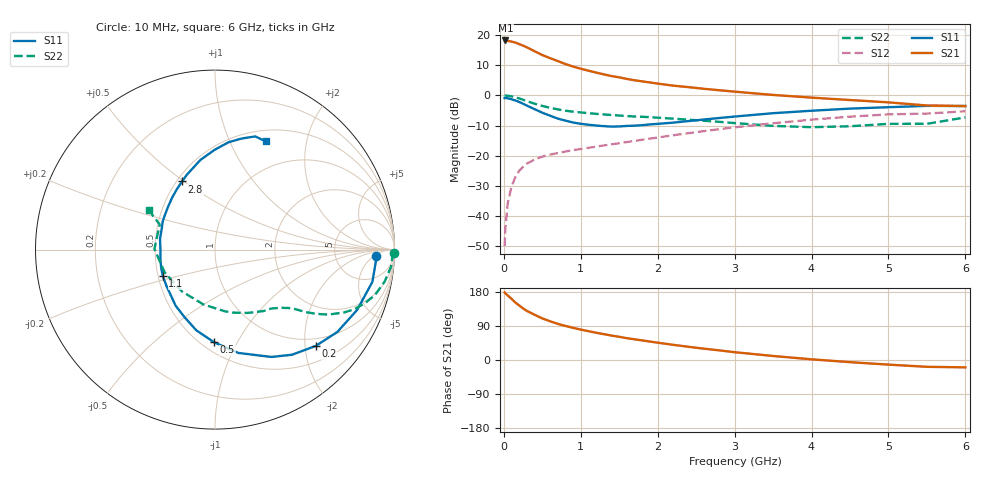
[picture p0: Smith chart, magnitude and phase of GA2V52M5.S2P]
! Infineon Technologies  Discrete & RF Semiconductors
! BF775
! Si NPN RF Bipolar Junction Transistor in SOT23
! VCE = 2.5 V  IC = 2.5 mA
! Common Emitter S-Parameters:  May  1996
# GHz  S  MA  R  50
!  f  S11  S21  S12  S22
! GHz  MAG  ANG  MAG  ANG  MAG  ANG  MAG  ANG
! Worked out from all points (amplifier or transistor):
!   36 points, 10 MHz to 6 GHz, reference 50 ohm
!   highest |S21| = 18.2 dB at 20 MHz (marker M1)
!   |S21| within 3 dB of that: start of sweep to 355.6 MHz
!   unconditionally stable (mu >= 1): 1.063 GHz to 3.976 GHz; 5.268 GHz to 5.979 GHz
!   at 250 MHz: K = 0.32, MSG = 20.0 dB, |S12| = -23.6 dB
!   at 1.4 GHz: K = 1.13, MAG = 9.1 dB, |S12| = -16.2 dB
!   at 6 GHz: K = 1.00, MSG = 0.9 dB, |S12| = -5.3 dB
!   S11 on the Smith chart (normalised r, x): 10 MHz: 16, -7; 200 MHz: 0.83, -2.23; 500 MHz: 0.57, -0.81; 1.1 GHz: 0.53, -0.18; 2.8 GHz: 0.53, +0.49; 6 GHz: 0.63, +1.37
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0.01  0.9003 -2.4  7.995 178.3  0.0032 88.0  0.9969 -1.0
0.02  0.8981 -4.6  8.082 176.0  0.0063 84.0  0.9895 -2.2
0.05  0.8951 -11.6  7.949 170.4  0.0162 83.3  0.9854 -5.6
0.1  0.8602 -23.0  7.75 161.4  0.031 77.0  0.9616 -10.7
0.15  0.8219 -33.9  7.457 151.5  0.0445 71.0  0.927 -15.8
0.2  0.7767 -43.7  7.034 143.9  0.0566 66.2  0.888 -19.6
0.25  0.726 -53.8  6.641 136.2  0.0658 62.0  0.8451 -23.1
0.3  0.6756 -62.3  6.213 129.5  0.0744 58.3  0.8014 -25.9
0.4  0.5901 -77.3  5.357 119.3  0.0868 53.0  0.7268 -29.9
0.5  0.5161 -90.6  4.635 109.8  0.0969 49.7  0.6682 -32.4
0.6  0.4609 -103.2  4.125 102.2  0.1046 47.7  0.622 -34.2
0.7  0.4126 -114.4  3.692 95.5  0.1109 46.7  0.586 -35.5
0.9  0.3555 -133.5  2.99 84.9  0.1241 45.8  0.5367 -37.5
1.1  0.3264 -152.9  2.555 76.0  0.1355 46.1  0.5069 -39.9
1.4  0.3039 -177.5  2.082 64.5  0.1545 47.0  0.4729 -43.6
1.6  0.312 168.9  1.865 57.5  0.1689 47.5  0.4537 -46.5
2.2  0.3533 137.9  1.446 40.1  0.2183 47.4  0.4114 -58.1
2.8  0.4216 115.8  1.214 25.4  0.2752 44.2  0.3646 -74.3
3.5  0.5064 99.2  1.015 10.6  0.3453 37.6  0.3123 -102.0
4.5  0.6029 82.8  0.836 -5.7  0.4436 25.1  0.3079 -155.7
5.5  0.6694 70.4  0.679 -18.0  0.499 9.7  0.3381 155.6
6  0.6658 65.0  0.664 -19.4  0.5451 5.5  0.4315 149.1
